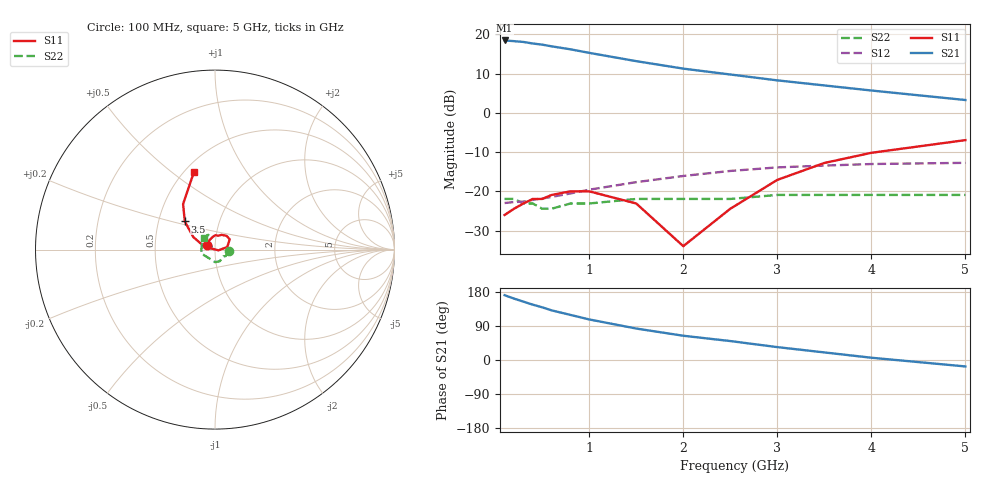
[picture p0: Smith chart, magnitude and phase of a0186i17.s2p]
!  MSA-0186 S AND NOISE PARAMETERS
!  Id=17mA  LAST UPDATED 07-22-92
# ghz s ma r 50
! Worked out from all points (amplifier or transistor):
!   15 points, 100 MHz to 5 GHz, reference 50 ohm
!   highest |S21| = 18.5 dB at 100 MHz (marker M1)
!   |S21| within 3 dB of that: start of sweep to 964.2 MHz
!   unconditionally stable (mu >= 1): start of sweep to end of sweep
!   at 300 MHz: K = 1.13, MAG = 18.2 dB, |S12| = -22.6 dB
!   at 1 GHz: K = 1.12, MAG = 15.4 dB, |S12| = -19.6 dB
!   at 5 GHz: K = 1.35, MAG = 4.5 dB, |S12| = -12.7 dB
!   lowest NFmin = 5.20 dB at 100 MHz
!   S11 on the Smith chart (normalised r, x): 100 MHz: 0.92, +0.05; 3.5 GHz: 0.68, +0.23; 5 GHz: 0.56, +0.61
0.1  0.05 148.0  8.39 171.0  0.071 4.0  0.08 -7.0
0.2  0.06 124.0  8.22 162.0  0.073 9.0  0.08 -14.0
0.3  0.07 103.0  8.03 154.0  0.074 13.0  0.07 -24.0
0.4  0.08 89.0  7.67 146.0  0.078 14.0  0.07 -31.0
0.5  0.08 76.0  7.42 139.0  0.081 17.0  0.06 -39.0
0.6  0.09 66.0  7.06 131.0  0.085 21.0  0.06 -47.0
0.8  0.1 50.0  6.47 119.0  0.094 25.0  0.07 -67.0
1  0.1 35.0  5.83 107.0  0.105 29.0  0.07 -89.0
1.5  0.07 12.0  4.57 83.0  0.131 30.0  0.08 -165.0
2  0.02 -12.0  3.67 64.0  0.157 27.0  0.08 156.0
2.5  0.06 165.0  3.09 50.0  0.182 24.0  0.08 134.0
3  0.14 150.0  2.6 34.0  0.202 19.0  0.09 124.0
3.5  0.23 137.0  2.24 20.0  0.213 12.0  0.09 117.0
4  0.31 125.0  1.93 6.0  0.223 5.0  0.09 114.0
5  0.45 105.0  1.46 -17.0  0.231 -5.0  0.09 132.0
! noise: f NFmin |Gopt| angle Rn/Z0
0.1  5.2  0.23  1  1.13
0.5  5.3  0.23  4  1.12
1  5.5  0.21  8  1.1
2  5.8  0.16  11  1.02
